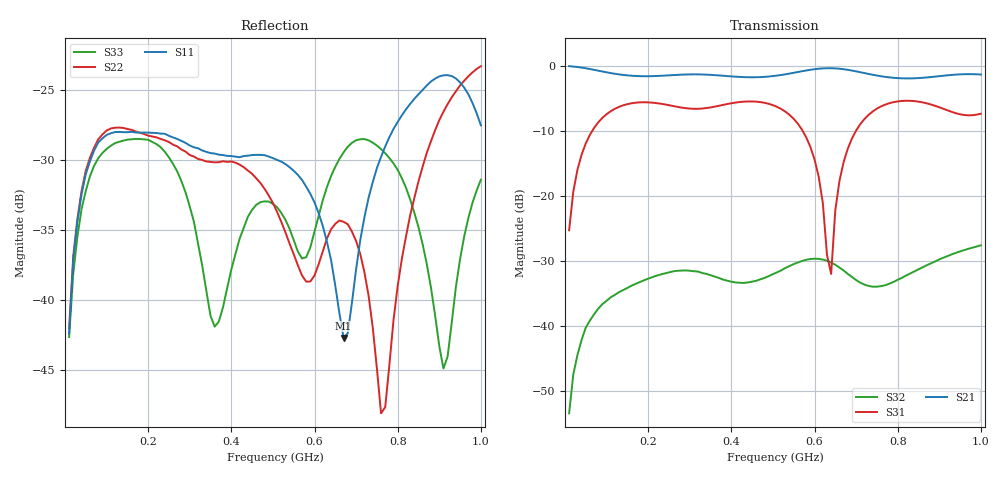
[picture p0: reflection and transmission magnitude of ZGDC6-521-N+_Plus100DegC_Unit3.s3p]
!Created: 04-01-2020 at 16:36:16
!Mini-Circuits
!S3P DATA File Format
!Type: Directional Coupler
!Port 1: (Input); Port 2: (Output); Port 3: (Couple)
!TEST CONDITIONS: Z:50 OHM SYSTEM, INPUT POWER = -10dBm, TEMP:100°C
!MODEL: ZGDC6-521-N+
!S/N: U3_100C
# MHZ S DB R 50
!Frequency
!  S11 dB  S11 DEG  S12 dB  S12 DEG  S13 dB  S13 DEG
!  S21 dB  S21 DEG  S22 dB  S22 DEG  S23 dB  S23 DEG
!  S31 dB  S31 DEG  S32 dB  S32 DEG  S33 dB  S33 DEG
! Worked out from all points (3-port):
!   100 points, 10 MHz to 1 GHz, reference 50 ohm
!   strongest paths, dB at 10 MHz, 260 MHz, 510 MHz, 760 MHz, 1 GHz:
!     S21: 0.0, -1.4, -1.5, -1.6, -1.3
!     S31: -25.3, -6.2, -6.3, -6.2, -7.3
!     S32: -53.4, -31.6, -31.7, -33.9, -27.6
!   lowest |S11| = -42.7 dB at 670 MHz (marker M1), VSWR 1.01, Z = 50.7 - j0.209 ohm
!   |S11| at or under -10 dB: start of sweep to end of sweep
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10  -42.37 62.6  -0.05 -7.5  -25.22 83.3
    -0.03 -7.5  -41.97 54.7  -53.12 -111.3
    -25.27 83.4  -53.43 -121.0  -42.62 52.2
130  -28.02 9.4  -1.30 -88.5  -6.29 14.8
     -1.30 -88.5  -27.71 -21.4  -34.80 86.9
     -6.29 14.8  -34.80 86.8  -28.73 6.5
280  -28.66 -14.7  -1.34 -179.8  -6.39 -34.8
     -1.34 -179.8  -29.27 -128.5  -31.50 -75.6
     -6.40 -34.8  -31.48 -75.9  -31.52 -46.5
510  -30.01 -31.9  -1.48 37.2  -6.29 -98.9
     -1.48 37.2  -33.72 -20.7  -31.71 106.4
     -6.29 -98.9  -31.73 106.3  -33.38 -46.8
640  -37.18 -48.4  -0.35 -51.0  -32.00 35.4
     -0.35 -51.0  -34.94 123.7  -30.22 -12.0
     -32.00 35.5  -30.25 -12.0  -31.15 106.4
670  -42.70 -16.3  -0.50 -72.9  -14.79 -9.7
     -0.50 -72.9  -34.42 85.9  -31.47 -37.7
     -14.78 -9.7  -31.46 -37.6  -29.47 74.3
760  -29.79 31.8  -1.58 -132.1  -6.22 -63.6
     -1.58 -132.1  -48.06 -48.1  -33.85 -81.5
     -6.22 -63.6  -33.86 -81.6  -29.24 15.0
840  -25.66 6.7  -1.90 -178.6  -5.41 -98.6
     -1.90 -178.6  -32.73 170.5  -31.59 -123.6
     -5.41 -98.6  -31.60 -123.7  -33.78 -29.5
910  -23.99 -24.6  -1.50 138.7  -6.59 -119.7
     -1.50 138.7  -26.58 136.9  -29.49 -172.6
     -6.59 -119.7  -29.49 -172.5  -44.87 -133.6
1000  -27.55 -90.1  -1.32 78.5  -7.34 -127.0
      -1.32 78.5  -23.34 97.5  -27.59 117.6
      -7.34 -127.0  -27.59 117.5  -31.42 106.4
